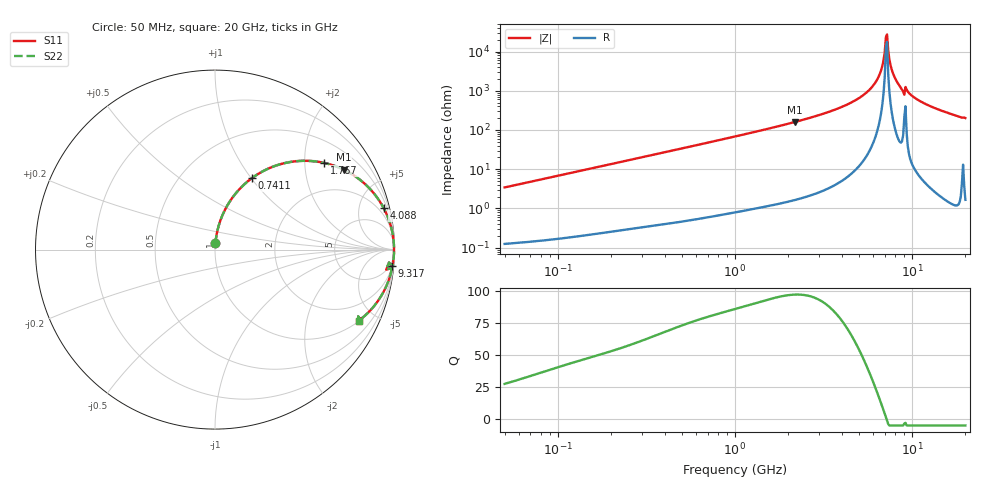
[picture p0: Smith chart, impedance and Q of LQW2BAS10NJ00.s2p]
!Murata Part Number: LQW2BAS10NJ00
!These Parameters are Measured in Series Mode Connection
!  o--[Z]--o
!Port1  Port2
!  o-------o
!Freq. Start=50[MHz] Stop=20[GHz], 401[Steps]
# Hz S RI R 50
!Freq.(Hz) S11(Real) S11(Imag) S21(Real) S21(Imag) S12(Real) S12(Imag) S22(Real) S22(Imag)
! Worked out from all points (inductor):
!   401 points, 50 MHz to 20 GHz, reference 50 ohm
!   read as one part in series: L = 10.9 nH near 51.52 MHz
!   highest Q = 97.3 at 2.179 GHz (marker M1), where L = 11.7 nH
!   self-resonance near 7.115 GHz
!   S11 on the Smith chart (normalised r, x): 50 MHz: 1.00, +0.07; 741.1 MHz: 1.01, +1.00; 1.767 GHz: 1.03, +2.51; 4.088 GHz: 1.11, +8.03; 9.317 GHz: 3, -21; 20 GHz: 1.03, -4.03
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5e7  0.00242 0.0342  0.9976 -0.0342  0.9976 -0.0342  0.00242 0.0342
1.364002e8  0.0105 0.0915  0.9895 -0.0915  0.9895 -0.0915  0.0105 0.0915
3.721004e8  0.0625 0.2346  0.9375 -0.2346  0.9375 -0.2346  0.0625 0.2346
7.411344e8  0.2042 0.397  0.7958 -0.397  0.7958 -0.397  0.2042 0.397
1e9  0.3194 0.4605  0.6806 -0.4605  0.6806 -0.4605  0.3194 0.4605
1.766834e9  0.6099 0.4826  0.3901 -0.4826  0.3901 -0.4826  0.6099 0.4826
2.179053e9  0.7165 0.4456  0.2835 -0.4456  0.2835 -0.4456  0.7165 0.4456
2.728004e9  0.8155 0.3827  0.1845 -0.3827  0.1845 -0.3827  0.8155 0.3827
4.087748e9  0.9389 0.233  0.0611 -0.233  0.0611 -0.233  0.9389 0.233
5.194772e9  0.9786 0.135  0.0214 -0.135  0.0214 -0.135  0.9786 0.135
6.125241e9  0.993 0.0664  0.00697 -0.0664  0.00697 -0.0664  0.993 0.0664
6.701223e9  0.9967 0.0288  0.00326 -0.0288  0.00326 -0.0288  0.9967 0.0288
7.009217e9  0.9975 0.00987  0.00249 -0.00987  0.00249 -0.00987  0.9975 0.00987
7.114996e9  0.9976 0.00354  0.0024 -0.00354  0.0024 -0.00354  0.9976 0.00354
7.331367e9  0.9975 -0.00915  0.00246 0.00915  0.00246 0.00915  0.9975 -0.00915
7.442007e9  0.9974 -0.0155  0.00261 0.0155  0.00261 0.0155  0.9974 -0.0155
7.668323e9  0.9968 -0.0283  0.00318 0.0283  0.00318 0.0283  0.9968 -0.0283
8.020766e9  0.9953 -0.0478  0.00473 0.0478  0.00473 0.0478  0.9953 -0.0478
8.774992e9  0.9869 -0.0922  0.0131 0.0922  0.0131 0.0922  0.9869 -0.0922
9.316812e9  0.9843 -0.0907  0.0157 0.0907  0.0157 0.0907  0.9843 -0.0907
1.257102e10  0.9422 -0.2292  0.0578 0.2292  0.0578 0.2292  0.9422 -0.2292
2e10  0.8006 -0.3954  0.1994 0.3954  0.1994 0.3954  0.8006 -0.3954
